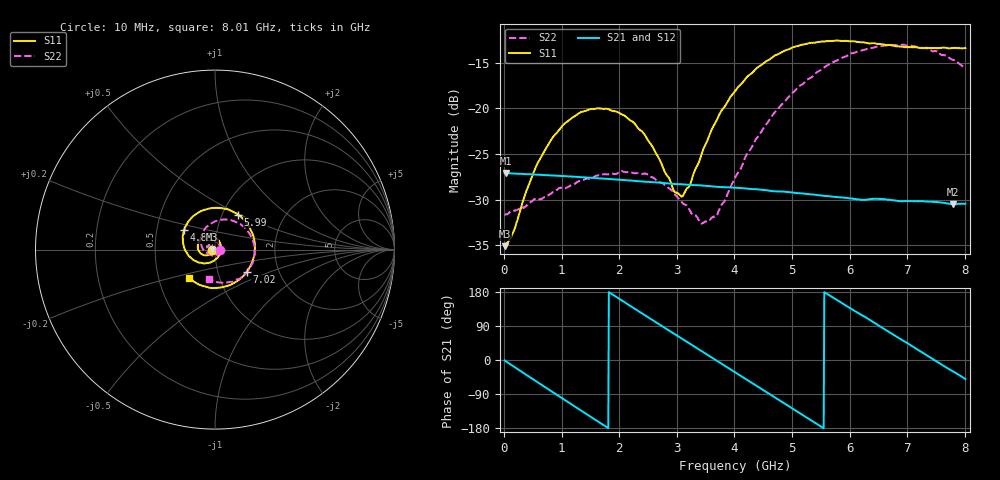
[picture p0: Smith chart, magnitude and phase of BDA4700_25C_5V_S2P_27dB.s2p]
!Agilent Technologies,E5071B,MY42404982,A.09.10
!Date: Mon Oct 20 13:40:06 2025
!Data & Calibration Information:
!Freq	S11:SOLT2(ON)	S21:SOLT2(ON)	S12:SOLT2(ON)	S22:SOLT2(ON)
# Hz S RI R 50
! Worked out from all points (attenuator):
!   801 points, 10 MHz to 8.01 GHz, reference 50 ohm
!   highest |S21| = -27.08 dB at 30 MHz (marker M1); lowest = -30.5 dB at 7.8 GHz (marker M2)
!   lowest |S11| = -35.1 dB at 10 MHz (marker M3), VSWR 1.04, Z = 48.3 - j0.0954 ohm
!   |S11| at or under -10 dB: start of sweep to end of sweep
!   |S22| runs from -32.6 to -13.0 dB; largest |S21 - S12| = 0.00038
!   S11 on the Smith chart (normalised r, x): 10 MHz: 0.97, -0.00; 4.83 GHz: 0.69, +0.16; 5.99 GHz: 1.18, +0.49; 7.02 GHz: 1.37, -0.36; 8.01 GHz: 0.72, -0.24
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1e7  -0.0175 -0.000988  0.0443 -0.000941  0.0443 -0.000993  0.0262 -0.000831
3e7  -0.0179 -0.00203  0.0442 -0.00246  0.0442 -0.00263  0.0262 -0.00157
7e8  -0.0484 -0.0323  0.0145 -0.0406  0.0145 -0.0406  0.00592 -0.0322
1.02e9  -0.0772 -0.023  -0.00888 -0.0416  -0.00893 -0.0416  -0.016 -0.033
1.35e9  -0.0955 0.00617  -0.0295 -0.0298  -0.0295 -0.0298  -0.0361 -0.0178
2.09e9  -0.05 0.0763  -0.0359 0.0185  -0.036 0.0186  -0.0292 0.0341
2.42e9  -0.00617 0.0731  -0.0202 0.0342  -0.0202 0.0342  -0.00493 0.0435
2.68e9  0.0215 0.0492  -0.00375 0.039  -0.00379 0.039  0.013 0.0374
2.95e9  0.0333 0.0117  0.0135 0.0361  0.0135 0.036  0.0253 0.0233
3.1e9  0.0309 -0.0114  0.022 0.0314  0.0219 0.0315  0.0281 0.0114
3.41e9  0.00373 -0.0533  0.0342 0.0162  0.0342 0.0162  0.0205 -0.0118
3.54e9  -0.0147 -0.0663  0.0366 0.00836  0.0366 0.00829  0.013 -0.0204
3.7e9  -0.044 -0.075  0.0371 -0.00159  0.0371 -0.00172  -0.000629 -0.0262
4.01e9  -0.1053 -0.0653  0.0311 -0.0196  0.0311 -0.0196  -0.0324 -0.0259
4.83e9  -0.1721 0.1091  -0.0126 -0.0326  -0.0125 -0.0327  -0.0772 0.0721
5.35e9  -0.071 0.2171  -0.0319 -0.011  -0.0319 -0.011  -0.0154 0.1482
5.99e9  0.128 0.1946  -0.0241 0.0214  -0.0242 0.0213  0.129 0.1483
6.68e9  0.2217 -0.0145  0.00871 0.0303  0.00877 0.0303  0.2203 0.000132
7.02e9  0.1756 -0.1261  0.0228 0.021  0.0229 0.021  0.2004 -0.0912
7.43e9  0.0531 -0.2067  0.0307 0.0021  0.0307 0.00203  0.1194 -0.1677
7.8e9  -0.0799 -0.1986  0.0256 -0.0152  0.0257 -0.0152  0.02 -0.1829
8.01e9  -0.1431 -0.1589  0.0192 -0.0231  0.0192 -0.023  -0.0309 -0.1624
